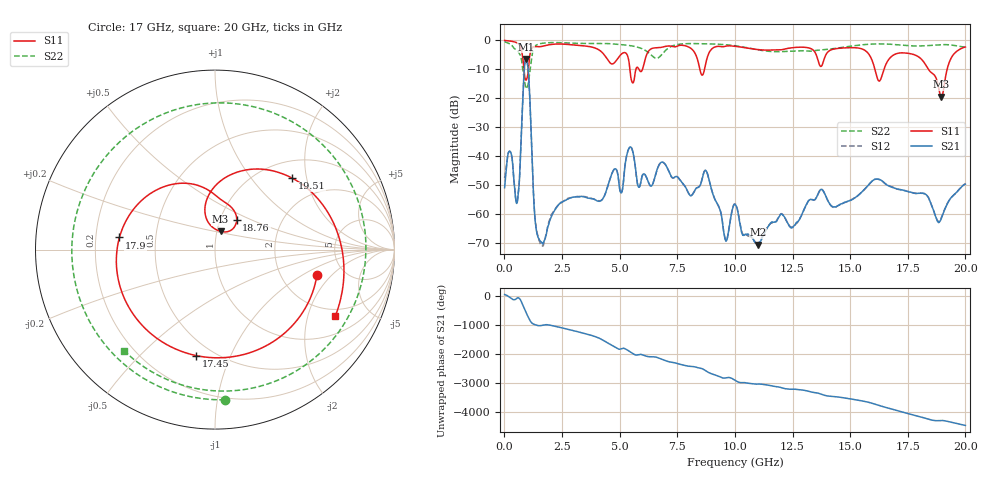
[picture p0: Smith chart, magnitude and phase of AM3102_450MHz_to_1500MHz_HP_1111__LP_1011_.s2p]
!Agilent Technologies,E8364B,MY43040894,A.07.50.67
!Agilent E8364B: A.07.50.67
!Date: Thursday, January 11, 2018 06:51:25
!Correction: S11(Full 2 Port(1,2))
!S21(Full 2 Port(1,2))
!S12(Full 2 Port(1,2))
!S22(Full 2 Port(1,2))
!S2P File: Measurements: S11, S21, S12, S22:
# Hz S  dB  R 50
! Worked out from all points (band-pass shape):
!   1601 points, 10 MHz to 20 GHz, reference 50 ohm
!   highest |S21| = -6.48 dB at 934.5 MHz (marker M1); lowest = -70.7 dB at 11 GHz (marker M2)
!   |S21| within 3 dB of the highest: 869 MHz to 1.023 GHz (154 MHz wide, 16.3 % of centre)
!   lowest |S11| = -19.5 dB at 18.95 GHz (marker M3), VSWR 1.24, Z = 52.1 + j10.7 ohm
!   |S11| at or under -10 dB: 5.444 GHz to 5.706 GHz (262.6 MHz wide, 4.71 % of centre); 16.07 GHz to 16.47 GHz (397.1 MHz wide, 2.44 % of centre); 18.39 GHz to 19.21 GHz (816 MHz wide, 4.34 % of centre)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
!   |S22| runs from -16.8 to -0.5 dB; largest |S21 - S12| = 0.0028
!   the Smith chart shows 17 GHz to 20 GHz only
!   S11 on the Smith chart (normalised r, x): 17 GHz: 3.17, -1.38; 17.45 GHz: 0.41, -0.75; 17.9 GHz: 0.30, +0.06; 18.76 GHz: 1.20, +0.41; 19.51 GHz: 1.36, +1.65; 20 GHz: 1.68, -3.01
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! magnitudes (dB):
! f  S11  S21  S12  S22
! 10 MHz  -0.1  -51.0  -47.6  -0.5
! 247.4 MHz  -0.3  -38.4  -38.4  -1.2
! 572.2 MHz  -1.0  -55.3  -55.1  -3.6
! 934.5 MHz  -13.8  -6.5  -6.5  -16.6
! 1.334 GHz  -2.2  -62.3  -61.8  -2.0
! 1.534 GHz  -2.2  -69.2  -69.7  -1.2
! 3.346 GHz  -1.9  -54.0  -54.1  -1.1
! 5.57 GHz  -14.7  -38.4  -38.5  -2.0
! 6.682 GHz  -2.6  -43.5  -43.6  -6.0
! 8.756 GHz  -7.3  -45.2  -45.2  -1.2
! 9.605 GHz  -2.0  -69.4  -69.1  -1.5
! 10.01 GHz  -2.1  -56.7  -56.6  -1.9
! 11 GHz  -3.2  -70.7  -70.3  -3.3
! 13.34 GHz  -3.1  -55.1  -55.1  -3.7
! 16.68 GHz  -6.6  -50.4  -50.3  -1.3
! 17 GHz  -4.7  -51.3  -51.3  -1.5
! 17.45 GHz  -4.4  -52.2  -52.1  -1.8
! 17.9 GHz  -5.4  -52.9  -52.9  -2.0
! 18.76 GHz  -13.8  -62.1  -62.0  -1.6
! 18.95 GHz  -19.5  -61.7  -61.5  -1.5
! 19.51 GHz  -4.6  -53.4  -53.4  -1.8
! 20 GHz  -2.3  -49.8  -49.5  -2.4
